FUNCTION_BLOCK FB_RemoveAllAxes //将轴移出轴组
VAR_INPUT
	Execute				: BOOL;
END_VAR
VAR_OUTPUT
	Done				: BOOL;
	Busy				: BOOL;
	Error				: BOOL;
END_VAR
VAR
	fbRemoveAxis			: ARRAY[1..4] OF MC_RemoveAxisFromGroup;
	i					: UINT;
END_VAR

Done := TRUE;
Busy := FALSE;
Error := FALSE;

fbRemoveAxis[1].IdentInGroup := MCS_X; //X-Axis
fbRemoveAxis[2].IdentInGroup := MCS_Y; //Y-Axis
fbRemoveAxis[3].IdentInGroup := MCS_Z; //Z-Axis
fbRemoveAxis[4].IdentInGroup := MCS_C1;//1st rotation is C-rotation (around Z-Axis)


fbRemoveAxis[1](AxesGroup:= stGroupRef , Execute:=Execute ,  );
fbRemoveAxis[2](AxesGroup:= stGroupRef , Execute:=Execute ,  );
fbRemoveAxis[3](AxesGroup:= stGroupRef , Execute:=Execute ,  );
fbRemoveAxis[4](AxesGroup:= stGroupRef , Execute:=Execute ,  );



FOR i:=1 TO 4 DO
	IF (NOT fbRemoveAxis[i].Done) THEN
		Done := FALSE;
	END_IF
	IF (fbRemoveAxis[i].Busy) THEN
		Busy := TRUE;
	END_IF
	IF (fbRemoveAxis[i].Error) THEN
		Error := TRUE;
	END_IF
END_FOR

END_FUNCTION_BLOCK
